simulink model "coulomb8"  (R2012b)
settings: Solver=ode2  StartTime=0.0  StopTime=100  FixedStep=0.001  MaxStep=0.001  RelTol=1e-3
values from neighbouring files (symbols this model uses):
  c = 2200    [coulomb_1.m]    (also in coulomb_10.m = 0.1; coulomb_11.m = 0; coulomb_2.m; coulomb_3.m)
  FG = 500    [coulomb_1.m]    (also in coulomb_10.m = 10; coulomb_11.m = 10; coulomb_2.m; coulomb_3.m)
  FH = 12    [coulomb_10.m]    (also in coulomb_11.m; coulomb_3.m = 600; coulomb_4.m = 600; position_reg_1.m = 3.956)
  k = 10    [coulomb_10.m]    (also in coulomb_11.m; diff_filter_1.m = 250; diff_filter_2.m = 250; dry_friction_1.m = 2200)
  m = 400    [coulomb_1.m]    (also in coulomb_10.m = 10; coulomb_11.m = 10; coulomb_2.m; coulomb_3.m)
  vstr = 0.1    [coulomb_10.m]    (also in coulomb_11.m; coulomb_3.m = 0.05; coulomb_4.m = 0.01; slip_stick_1.m = 0.01)
undefined symbols (not defined in the file or in its folder): sgn

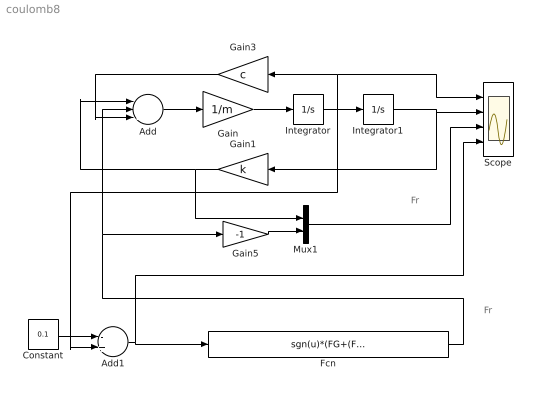
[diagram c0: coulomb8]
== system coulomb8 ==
  note: Fr
  note: Fr
  Add : Sum  Inputs=---
  Add1 : Sum  Inputs=-+
  Constant : Constant  Value=0.1
  Fcn : Fcn  Expr=sgn(u)*(FG+(FH-FG)*exp(-abs(u/vstr)))
  Gain : Gain  Gain=1/m
  Gain1 : Gain  Gain=k
  Gain3 : Gain  Gain=c
  Gain5 : Gain  Gain=-1
  Integrator : Integrator
  Integrator1 : Integrator
  Mux1 : Mux  Inputs=2
  Scope : Scope  NumInputPorts=4
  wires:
  Add/1 -> Gain/1
  Gain/1 -> Integrator/1
  Integrator1/1 -> Gain1/1, Scope/2
  Constant/1 -> Add1/1
  Integrator/1 -> Add1/2, Integrator1/1, Scope/1, Gain3/1
  Gain3/1 -> Add/3
  Gain1/1 -> Mux1/1, Add/1
  Mux1/1 -> Scope/3
  Add1/1 -> Fcn/1, Scope/4
  Gain5/1 -> Mux1/2
  Fcn/1 -> Gain5/1, Add/2
